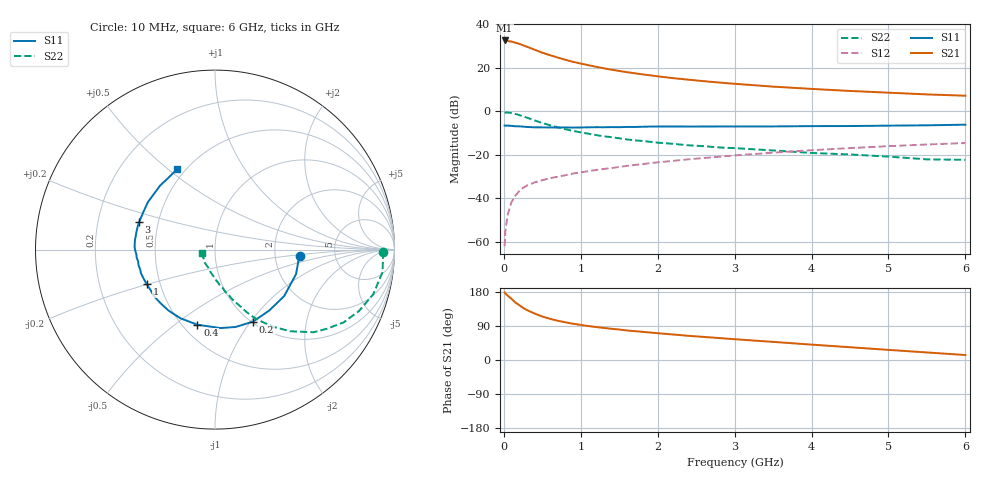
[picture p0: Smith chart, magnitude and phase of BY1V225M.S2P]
! SIEMENS Small Signal Semiconductors
! BFY420
! Si NPN RF SIEGET Grounded Emitter Transistor in MICRO-X
! VCE = 1.25 V  IC = 25 mA
! Common Emitter S-Parameters:  October  1996
# GHz  S  MA  R  50
!  f  S11  S21  S12  S22
! GHz  MAG  ANG  MAG  ANG  MAG  ANG  MAG  ANG
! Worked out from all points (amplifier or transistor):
!   36 points, 10 MHz to 6 GHz, reference 50 ohm
!   highest |S21| = 32.6 dB at 10 MHz (marker M1)
!   |S21| within 3 dB of that: start of sweep to 308.5 MHz
!   unconditionally stable (mu >= 1): start of sweep to 11.77 MHz; 1.625 GHz to end of sweep
!   at 250 MHz: K = 0.35, MSG = 32.8 dB, |S12| = -35.1 dB
!   at 1.4 GHz: K = 0.96, MSG = 22.6 dB, |S12| = -26.0 dB
!   at 6 GHz: K = 1.09, MAG = 9.1 dB, |S12| = -14.6 dB
!   S11 on the Smith chart (normalised r, x): 10 MHz: 2.78, -0.25; 200 MHz: 1.01, -1.03; 400 MHz: 0.59, -0.61; 1 GHz: 0.42, -0.20; 3 GHz: 0.39, +0.15; 6 GHz: 0.45, +0.54
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0.01  0.4743 -4.2  42.55 178.6  0.0008 111.9  0.9374 -0.7
0.02  0.469 -7.4  42.24 175.4  0.0018 99.9  0.9367 -2.4
0.1  0.4644 -33.9  40.12 161.3  0.0083 79.0  0.916 -15.8
0.15  0.4543 -48.4  37.82 151.8  0.0116 72.8  0.8722 -23.1
0.2  0.4537 -62.2  35.59 144.8  0.0147 68.1  0.8235 -29.5
0.25  0.4462 -75.0  32.98 137.6  0.0175 64.8  0.7654 -35.1
0.3  0.4382 -86.0  30.53 131.8  0.0198 62.8  0.7164 -40.0
0.4  0.4299 -103.2  26.11 122.6  0.0233 59.5  0.619 -47.3
0.5  0.4284 -116.8  22.29 114.7  0.0262 57.7  0.5411 -52.8
0.6  0.4272 -127.2  19.51 108.7  0.0293 56.8  0.479 -57.0
0.7  0.4259 -135.6  17.24 103.6  0.0314 57.2  0.4304 -60.5
0.8  0.4278 -142.6  15.31 99.4  0.0341 56.3  0.3884 -63.3
1  0.4265 -153.0  12.52 92.6  0.0397 57.2  0.3296 -67.3
1.1  0.4302 -158.7  11.5 89.6  0.0423 57.2  0.3065 -69.7
1.4  0.4348 -168.5  9.039 82.4  0.0499 57.6  0.2548 -74.5
1.6  0.4391 -174.3  7.94 78.0  0.0559 57.2  0.2271 -77.8
2.2  0.4493 173.1  5.797 67.3  0.0729 55.1  0.1797 -85.9
3  0.4499 159.9  4.3 54.9  0.0973 50.4  0.1431 -95.2
3.5  0.4509 151.9  3.701 47.8  0.1124 47.0  0.1265 -101.8
4.5  0.4602 137.8  2.944 33.7  0.1433 38.1  0.1023 -115.0
5.5  0.4779 122.4  2.452 19.9  0.1734 28.3  0.079 -144.8
6  0.4947 115.4  2.288 13.1  0.1872 23.3  0.077 -165.7
